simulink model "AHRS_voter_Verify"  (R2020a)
settings: Solver=FixedStepDiscrete  StartTime=0.0  StopTime=10.0  FixedStep=0.01  RelTol=1e-3
undefined symbols (not defined in the file or in its folder): sldvsubsys
libraries: sldvlib x1

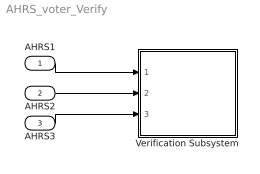
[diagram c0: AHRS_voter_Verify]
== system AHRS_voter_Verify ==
  AHRS1 : Inport  OutDataTypeStr=Bus: AHRS_Bus  PortDimensions=1  SampleTime=0.01
  AHRS2 : Inport  Port=2  OutDataTypeStr=Bus: AHRS_Bus  PortDimensions=1  SampleTime=0.01
  AHRS3 : Inport  Port=3  OutDataTypeStr=Bus: AHRS_Bus  PortDimensions=1  SampleTime=0.01
  Verification Subsystem : Subsystem  Tag=VerificationSubsystem  DisableCoverage=on  LoadFcn=sldvsubsys('check')  TreatAsAtomicUnit=on  SimViewingDevice=on  mask(VerificationSubsystem){}
      mask init:
      | sldvsubsys('maskInit');
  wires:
  AHRS1/1 -> Verification Subsystem/1(AHRS1)
  AHRS2/1 -> Verification Subsystem/2(AHRS2)
  AHRS3/1 -> Verification Subsystem/3(AHRS3)

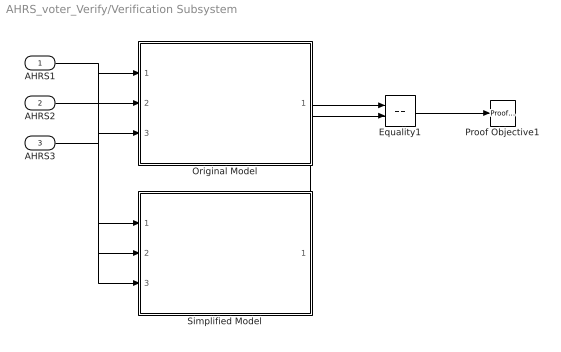
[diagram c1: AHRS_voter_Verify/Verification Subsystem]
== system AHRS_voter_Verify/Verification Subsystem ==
  AHRS1 : Inport  OutDataTypeStr=Bus: AHRS_Bus  PortDimensions=1  SampleTime=0.01
  AHRS2 : Inport  Port=2  OutDataTypeStr=Bus: AHRS_Bus  PortDimensions=1  SampleTime=0.01
  AHRS3 : Inport  Port=3  OutDataTypeStr=Bus: AHRS_Bus  PortDimensions=1  SampleTime=0.01
  Equality1 : RelationalOperator  Operator===  OutDataTypeStr=boolean  RndMeth=Simplest
  Original Model : ModelReference  ModelNameDialog=AHRS_voter_Original  SimulationMode=Normal  ModelReferenceVersion=1.74
  Proof Objective1 : sldvlib/Objectives and Constraints/Proof Objective  enabled=on  customAVTBlockType=Proof Objective  intervals=true  dispValues=on  outEnabled=off  enableStopSim=off
  Simplified Model : ModelReference  ModelNameDialog=AHRS_voter_New  SimulationMode=Normal  ModelReferenceVersion=1.80
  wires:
  AHRS1/1 -> Original Model/1, Simplified Model/1
  AHRS2/1 -> Original Model/2, Simplified Model/2
  AHRS3/1 -> Original Model/3, Simplified Model/3
  Original Model/1 -> Equality1/1
  Simplified Model/1 -> Equality1/2
  Equality1/1 -> Proof Objective1/1
